TYPE STR_HEATER_FURNACE :
STRUCT
//INPUT
	Input_LOOP1_Process_Value	AT%I*	:	REAL	;
	Input_LOOP1_Alarm_Condition	AT%I*	:	UINT	;
	Input_LOOP1_Manipulated_Value_Control_Output	AT%I*	:	REAL	;
	Input_LOOP1_Controlling_Set_Point	AT%I*	:	REAL	;
	Input_LOOP1_Actual_Control_State	AT%I*	:	BOOL	;
	Input_LOOP1_Sensor_Error	AT%I*	:	BOOL	;
	Input_LOOP1_Actual_Control_Loop_Mode	AT%I*	:	BOOL	;
	Input_LOOP2_Process_Value	AT%I*	:	REAL	;
	Input_LOOP2_Alarm_Condition	AT%I*	:	UINT	;
	Input_LOOP2_Manipulated_Value_Control_Output	AT%I*	:	REAL	;
	Input_LOOP2_Controlling_Set_Point	AT%I*	:	REAL	;
	Input_LOOP2_Actual_Control_State	AT%I*	:	BOOL	;
	Input_LOOP2_Sensor_Error	AT%I*	:	BOOL	;
	Input_LOOP2_Actual_Control_Loop_Mode	AT%I*	:	BOOL	;
	Input_LOOP3_Process_Value	AT%I*	:	REAL	;
	Input_LOOP3_Alarm_Condition	AT%I*	:	UINT	;
	Input_LOOP3_Manipulated_Value_Control_Output	AT%I*	:	REAL	;
	Input_LOOP3_Controlling_Set_Point	AT%I*	:	REAL	;
	Input_LOOP3_Actual_Control_State	AT%I*	:	BOOL	;
	Input_LOOP3_Sensor_Error	AT%I*	:	BOOL	;
	Input_LOOP3_Actual_Control_Loop_Mode	AT%I*	:	BOOL	;
	Input_LOOP4_Process_Value	AT%I*	:	REAL	;
	Input_LOOP4_Alarm_Condition	AT%I*	:	UINT	;
	Input_LOOP4_Manipulated_Value_Control_Output	AT%I*	:	REAL	;
	Input_LOOP4_Controlling_Set_Point	AT%I*	:	REAL	;
	Input_LOOP4_Actual_Control_State	AT%I*	:	BOOL	;
	Input_LOOP4_Sensor_Error	AT%I*	:	BOOL	;
	Input_LOOP4_Actual_Control_Loop_Mode	AT%I*	:	BOOL	;
	Input_LOOP5_Process_Value	AT%I*	:	REAL	;
	Input_LOOP5_Alarm_Condition	AT%I*	:	UINT	;
	Input_LOOP5_Manipulated_Value_Control_Output	AT%I*	:	REAL	;
	Input_LOOP5_Controlling_Set_Point	AT%I*	:	REAL	;
	Input_LOOP5_Actual_Control_State	AT%I*	:	BOOL	;
	Input_LOOP5_Sensor_Error	AT%I*	:	BOOL	;
	Input_LOOP5_Actual_Control_Loop_Mode	AT%I*	:	BOOL	;
	Input_LOOP6_Process_Value	AT%I*	:	REAL	;
	Input_LOOP6_Alarm_Condition	AT%I*	:	UINT	;
	Input_LOOP6_Manipulated_Value_Control_Output	AT%I*	:	REAL	;
	Input_LOOP6_Controlling_Set_Point	AT%I*	:	REAL	;
	Input_LOOP6_Actual_Control_State	AT%I*	:	BOOL	;
	Input_LOOP6_Sensor_Error	AT%I*	:	BOOL	;
	Input_LOOP6_Actual_Control_Loop_Mode	AT%I*	:	BOOL	;
	Input_LOOP7_Process_Value	AT%I*	:	REAL	;
	Input_LOOP7_Alarm_Condition	AT%I*	:	UINT	;
	Input_LOOP7_Manipulated_Value_Control_Output	AT%I*	:	REAL	;
	Input_LOOP7_Controlling_Set_Point	AT%I*	:	REAL	;
	Input_LOOP7_Actual_Control_State	AT%I*	:	BOOL	;
	Input_LOOP7_Sensor_Error	AT%I*	:	BOOL	;
	Input_LOOP7_Actual_Control_Loop_Mode	AT%I*	:	BOOL	;
	Input_LOOP8_Process_Value	AT%I*	:	REAL	;
	Input_LOOP8_Alarm_Condition	AT%I*	:	UINT	;
	Input_LOOP8_Manipulated_Value_Control_Output	AT%I*	:	REAL	;
	Input_LOOP8_Controlling_Set_Point	AT%I*	:	REAL	;
	Input_LOOP8_Actual_Control_State	AT%I*	:	BOOL	;
	Input_LOOP8_Sensor_Error	AT%I*	:	BOOL	;
	Input_LOOP8_Actual_Control_Loop_Mode	AT%I*	:	BOOL	;
	Input_IO_Mod_1_PV	AT%I*	:	REAL	;
	Input_IO_Mod_2_PV	AT%I*	:	REAL	;
	Input_IO_Mod_3_PV	AT%I*	:	REAL	;
	Input_IO_Mod_4_PV	AT%I*	:	REAL	;
	Input_IO_Mod_5_PV	AT%I*	:	REAL	;
	Input_IO_Mod_6_PV	AT%I*	:	REAL	;
	Input_IO_Mod_7_PV	AT%I*	:	REAL	;
	Input_IO_Mod_9_PV	AT%I*	:	REAL	;
	Input_IO_Mod_10_PV	AT%I*	:	REAL	;
	Input_IO_Mod_11_PV	AT%I*	:	REAL	;
	Input_IO_Mod_12_PV	AT%I*	:	REAL	;
	Input_IO_Mod_13_PV	AT%I*	:	REAL	;
	Input_IO_Mod_14_PV	AT%I*	:	REAL	;
	Input_IO_Mod_15_PV	AT%I*	:	REAL	;
	Input_IO_Mod_18_PV	AT%I*	:	REAL	;
	Input_IO_Mod_19_PV	AT%I*	:	REAL	;
	Input_IO_Mod_20_PV	AT%I*	:	REAL	;
	Input_IO_Mod_21_PV	AT%I*	:	REAL	;
	Input_IO_Mod_22_PV	AT%I*	:	REAL	;
	Input_IO_Mod_23_PV	AT%I*	:	REAL	;
	Input_IO_Mod_1_SBrkOut	AT%I*	:	USINT	;
	Input_IO_Mod_2_SBrkOut	AT%I*	:	USINT	;
	Input_IO_Mod_3_SBrkOut	AT%I*	:	USINT	;
	Input_IO_Mod_4_SBrkOut	AT%I*	:	USINT	;
	Input_IO_Mod_5_SBrkOut	AT%I*	:	USINT	;
	Input_IO_Mod_6_SBrkOut	AT%I*	:	USINT	;
	Input_IO_Mod_7_SBrkOut	AT%I*	:	USINT	;
	Input_IO_Mod_9_SBrkOut	AT%I*	:	USINT	;
	Input_IO_Mod_10_SBrkOut	AT%I*	:	USINT	;
	Input_IO_Mod_11_SBrkOut	AT%I*	:	USINT	;
	Input_IO_Mod_12_SBrkOut	AT%I*	:	USINT	;
	Input_IO_Mod_13_SBrkOut	AT%I*	:	USINT	;
	Input_IO_Mod_14_SBrkOut	AT%I*	:	USINT	;
	Input_IO_Mod_15_SBrkOut	AT%I*	:	USINT	;
	Input_IO_Mod_18_SBrkOut	AT%I*	:	USINT	;
	Input_IO_Mod_19_SBrkOut	AT%I*	:	USINT	;
	Input_IO_Mod_20_SBrkOut	AT%I*	:	USINT	;
	Input_IO_Mod_21_SBrkOut	AT%I*	:	USINT	;
	Input_IO_Mod_22_SBrkOut	AT%I*	:	USINT	;
	Input_IO_Mod_23_SBrkOut	AT%I*	:	USINT	;
	Input_Math2_8_In2	AT%I*	:	REAL	;
	Input_Math2_12_In2	AT%I*	:	REAL	;
	Input_Math2_16_In2	AT%I*	:	REAL	;
	Input_Math2_20_In2	AT%I*	:	REAL	;
	Input_Math2_24_In2	AT%I*	:	REAL	;
	Input_Math2_28_In2	AT%I*	:	REAL	;
	Input_Loop_7_Setpoint	AT%I*	:	REAL	;
	Input_Loop_7_Setpoint_SPRateUp	AT%I*	:	REAL	;
	Input_Loop_7_Setpoint_SPRateDown	AT%I*	:	REAL	;
	Input_Loop_7_PID_Ch1PropBand	AT%I*	:	REAL	;
	Input_Loop_7_PID_IntegralTime	AT%I*	:	REAL	;
	Input_Loop_7_PID_DerivativeTime	AT%I*	:	REAL	;
	Input_Loop_1_Main_CascadeMode	AT%I*	:	USINT	;
	Input_Loop_1_Setpoint	AT%I*	:	REAL	;
	Input_Loop_1_Setpoint_SPRateUp	AT%I*	:	REAL	;
	Input_Loop_1_Setpoint_SPRateDown	AT%I*	:	REAL	;
	Input_Loop_1_Cascade_SecondaryLocalSP	AT%I*	:	REAL	;
	Input_Loop_1_Main_TC_Select	AT%I*	:	USINT	;
	Input_Loop_1_PrimaryPID_PrimaryPropBand	AT%I*	:	REAL	;
	Input_Loop_1_PrimaryPID_PrimaryIntegralTime	AT%I*	:	REAL	;
	Input_Loop_1_PrimaryPID_PrimaryDerivativeTime	AT%I*	:	REAL	;
	Input_Loop_1_PID_Ch1PropBand	AT%I*	:	REAL	;
	Input_Loop_1_PID_IntegralTime	AT%I*	:	REAL	;
	Input_Loop_1_PID_DerivativeTime	AT%I*	:	REAL	;
	Input_Loop_2_Main_CascadeMode	AT%I*	:	USINT	;
	Input_Loop_2_Setpoint	AT%I*	:	REAL	;
	Input_Loop_2_Setpoint_SPRateUp	AT%I*	:	REAL	;
	Input_Loop_2_Setpoint_SPRateDown	AT%I*	:	REAL	;
	Input_Loop_2_Cascade_SecondaryLocalSP	AT%I*	:	REAL	;
	Input_Loop_2_Main_TC_Select	AT%I*	:	USINT	;
	Input_Loop_2_PrimaryPID_PrimaryPropBand	AT%I*	:	REAL	;
	Input_Loop_2_PrimaryPID_PrimaryIntegralTime	AT%I*	:	REAL	;
	Input_Loop_2_PrimaryPID_PrimaryDerivativeTime	AT%I*	:	REAL	;
	Input_Loop_2_PID_Ch1PropBand	AT%I*	:	REAL	;
	Input_Loop_2_PID_IntegralTime	AT%I*	:	REAL	;
	Input_Loop_2_PID_DerivativeTime	AT%I*	:	REAL	;
	Input_Loop_3_Main_CascadeMode	AT%I*	:	USINT	;
	Input_Loop_3_Setpoint	AT%I*	:	REAL	;
	Input_Loop_3_Setpoint_SPRateUp	AT%I*	:	REAL	;
	Input_Loop_3_Setpoint_SPRateDown	AT%I*	:	REAL	;
	Input_Loop_3_Cascade_SecondaryLocalSP	AT%I*	:	REAL	;
	Input_Loop_3_Main_TC_Select	AT%I*	:	USINT	;
	Input_Loop_3_PrimaryPID_PrimaryPropBand	AT%I*	:	REAL	;
	Input_Loop_3_PrimaryPID_PrimaryIntegralTime	AT%I*	:	REAL	;
	Input_Loop_3_PrimaryPID_PrimaryDerivativeTime	AT%I*	:	REAL	;
	Input_Loop_3_PID_Ch1PropBand	AT%I*	:	REAL	;
	Input_Loop_3_PID_IntegralTime	AT%I*	:	REAL	;
	Input_Loop_3_PID_DerivativeTime	AT%I*	:	REAL	;
	Input_Loop_4_Main_CascadeMode	AT%I*	:	USINT	;
	Input_Loop_4_Setpoint	AT%I*	:	REAL	;
	Input_Loop_4_Setpoint_SPRateUp	AT%I*	:	REAL	;
	Input_Loop_4_Setpoint_SPRateDown	AT%I*	:	REAL	;
	Input_Loop_4_Cascade_SecondaryLocalSP	AT%I*	:	REAL	;
	Input_Loop_4_Main_TC_Select	AT%I*	:	USINT	;
	Input_Loop_4_PrimaryPID_PrimaryPropBand	AT%I*	:	REAL	;
	Input_Loop_4_PrimaryPID_PrimaryIntegralTime	AT%I*	:	REAL	;
	Input_Loop_4_PrimaryPID_PrimaryDerivativeTime	AT%I*	:	REAL	;
	Input_Loop_4_PID_Ch1PropBand	AT%I*	:	REAL	;
	Input_Loop_4_PID_IntegralTime	AT%I*	:	REAL	;
	Input_Loop_4_PID_DerivativeTime	AT%I*	:	REAL	;
	Input_Loop_5_Main_CascadeMode	AT%I*	:	USINT	;
	Input_Loop_5_Setpoint	AT%I*	:	REAL	;
	Input_Loop_5_Setpoint_SPRateUp	AT%I*	:	REAL	;
	Input_Loop_5_Setpoint_SPRateDown	AT%I*	:	REAL	;
	Input_Loop_5_Cascade_SecondaryLocalSP	AT%I*	:	REAL	;
	Input_Loop_5_Main_TC_Select	AT%I*	:	USINT	;
	Input_Loop_5_PrimaryPID_PrimaryPropBand	AT%I*	:	REAL	;
	Input_Loop_5_PrimaryPID_PrimaryIntegralTime	AT%I*	:	REAL	;
	Input_Loop_5_PrimaryPID_PrimaryDerivativeTime	AT%I*	:	REAL	;
	Input_Loop_5_PID_Ch1PropBand	AT%I*	:	REAL	;
	Input_Loop_5_PID_IntegralTime	AT%I*	:	REAL	;
	Input_Loop_5_PID_DerivativeTime	AT%I*	:	REAL	;
	Input_Loop_6_Main_CascadeMode	AT%I*	:	USINT	;
	Input_Loop_6_Setpoint	AT%I*	:	REAL	;
	Input_Loop_6_Setpoint_SPRateUp	AT%I*	:	REAL	;
	Input_Loop_6_Setpoint_SPRateDown	AT%I*	:	REAL	;
	Input_Loop_6_Cascade_SecondaryLocalSP	AT%I*	:	REAL	;
	Input_Loop_6_Main_TC_Select	AT%I*	:	USINT	;
	Input_Loop_6_PrimaryPID_PrimaryPropBand	AT%I*	:	REAL	;
	Input_Loop_6_PrimaryPID_PrimaryIntegralTime	AT%I*	:	REAL	;
	Input_Loop_6_PrimaryPID_PrimaryDerivativeTime	AT%I*	:	REAL	;
	Input_Loop_6_PID_Ch1PropBand	AT%I*	:	REAL	;
	Input_Loop_6_PID_IntegralTime	AT%I*	:	REAL	;
	Input_Loop_6_PID_DerivativeTime	AT%I*	:	REAL	;
	Input_Instrument_Diagnostics_ForceStandby	AT%I*	:	USINT	;
	
//OUTPUT
	Output_LOOP1_Target_Set_Point	AT%Q*	:	REAL	;
	Output_LOOP1_Clear_Alarms	AT%Q*	:	UINT	;
	Output_LOOP1_Forced_MV	AT%Q*	:	REAL	;
	Output_LOOP1_Control_Mode	AT%Q*	:	BOOL	;
	Output_LOOP1_Control_State	AT%Q*	:	BOOL	;
	Output_LOOP2_Target_Set_Point	AT%Q*	:	REAL	;
	Output_LOOP2_Clear_Alarms	AT%Q*	:	UINT	;
	Output_LOOP2_Forced_MV	AT%Q*	:	REAL	;
	Output_LOOP2_Control_Mode	AT%Q*	:	BOOL	;
	Output_LOOP2_Control_State	AT%Q*	:	BOOL	;
	Output_LOOP3_Target_Set_Point	AT%Q*	:	REAL	;
	Output_LOOP3_Clear_Alarms	AT%Q*	:	UINT	;
	Output_LOOP3_Forced_MV	AT%Q*	:	REAL	;
	Output_LOOP3_Control_Mode	AT%Q*	:	BOOL	;
	Output_LOOP3_Control_State	AT%Q*	:	BOOL	;
	Output_LOOP4_Target_Set_Point	AT%Q*	:	REAL	;
	Output_LOOP4_Clear_Alarms	AT%Q*	:	UINT	;
	Output_LOOP4_Forced_MV	AT%Q*	:	REAL	;
	Output_LOOP4_Control_Mode	AT%Q*	:	BOOL	;
	Output_LOOP4_Control_State	AT%Q*	:	BOOL	;
	Output_LOOP5_Target_Set_Point	AT%Q*	:	REAL	;
	Output_LOOP5_Clear_Alarms	AT%Q*	:	UINT	;
	Output_LOOP5_Forced_MV	AT%Q*	:	REAL	;
	Output_LOOP5_Control_Mode	AT%Q*	:	BOOL	;
	Output_LOOP5_Control_State	AT%Q*	:	BOOL	;
	Output_LOOP6_Target_Set_Point	AT%Q*	:	REAL	;
	Output_LOOP6_Clear_Alarms	AT%Q*	:	UINT	;
	Output_LOOP6_Forced_MV	AT%Q*	:	REAL	;
	Output_LOOP6_Control_Mode	AT%Q*	:	BOOL	;
	Output_LOOP6_Control_State	AT%Q*	:	BOOL	;
	Output_LOOP7_Target_Set_Point	AT%Q*	:	REAL	;
	Output_LOOP7_Clear_Alarms	AT%Q*	:	UINT	;
	Output_LOOP7_Forced_MV	AT%Q*	:	REAL	;
	Output_LOOP7_Control_Mode	AT%Q*	:	BOOL	;
	Output_LOOP7_Control_State	AT%Q*	:	BOOL	;
	Output_LOOP8_Target_Set_Point	AT%Q*	:	REAL	;
	Output_LOOP8_Clear_Alarms	AT%Q*	:	UINT	;
	Output_LOOP8_Forced_MV	AT%Q*	:	REAL	;
	Output_LOOP8_Control_Mode	AT%Q*	:	BOOL	;
	Output_LOOP8_Control_State	AT%Q*	:	BOOL	;
	Output_Math2_8_In2	AT%Q*	:	REAL	;
	Output_Math2_12_In2	AT%Q*	:	REAL	;
	Output_Math2_16_In2	AT%Q*	:	REAL	;
	Output_Math2_20_In2	AT%Q*	:	REAL	;
	Output_Math2_24_In2	AT%Q*	:	REAL	;
	Output_Math2_28_In2	AT%Q*	:	REAL	;
	Output_Loop_7_Setpoint_SPRateUp	AT%Q*	:	REAL	;
	Output_Loop_7_Setpoint_SPRateDown	AT%Q*	:	REAL	;
	Output_Loop_7_PID_Ch1PropBand	AT%Q*	:	REAL	;
	Output_Loop_7_PID_IntegralTime	AT%Q*	:	REAL	;
	Output_Loop_7_PID_DerivativeTime	AT%Q*	:	REAL	;
	Output_Loop_1_Main_CascadeMode	AT%Q*	:	USINT	;
	Output_Loop_1_Setpoint_SPRateUp	AT%Q*	:	REAL	;
	Output_Loop_1_Setpoint_SPRateDown	AT%Q*	:	REAL	;
	Output_Loop_1_Cascade_SecondaryLocalSP	AT%Q*	:	REAL	;
	Output_Loop_1_Main_TC_Select	AT%Q*	:	USINT	;
	Output_Loop_1_PrimaryPID_PrimaryPropBand	AT%Q*	:	REAL	;
	Output_Loop_1_PrimaryPID_PrimaryIntegralTime	AT%Q*	:	REAL	;
	Output_Loop_1_PrimaryPID_PrimaryDerivativeTime	AT%Q*	:	REAL	;
	Output_Loop_1_PID_Ch1PropBand	AT%Q*	:	REAL	;
	Output_Loop_1_PID_IntegralTime	AT%Q*	:	REAL	;
	Output_Loop_1_PID_DerivativeTime	AT%Q*	:	REAL	;
	Output_Loop_2_Main_CascadeMode	AT%Q*	:	USINT	;
	Output_Loop_2_Setpoint_SPRateUp	AT%Q*	:	REAL	;
	Output_Loop_2_Setpoint_SPRateDown	AT%Q*	:	REAL	;
	Output_Loop_2_Cascade_SecondaryLocalSP	AT%Q*	:	REAL	;
	Output_Loop_2_Main_TC_Select	AT%Q*	:	USINT	;
	Output_Loop_2_PrimaryPID_PrimaryPropBand	AT%Q*	:	REAL	;
	Output_Loop_2_PrimaryPID_PrimaryIntegralTime	AT%Q*	:	REAL	;
	Output_Loop_2_PrimaryPID_PrimaryDerivativeTime	AT%Q*	:	REAL	;
	Output_Loop_2_PID_Ch1PropBand	AT%Q*	:	REAL	;
	Output_Loop_2_PID_IntegralTime	AT%Q*	:	REAL	;
	Output_Loop_2_PID_DerivativeTime	AT%Q*	:	REAL	;
	Output_Loop_3_Main_CascadeMode	AT%Q*	:	USINT	;
	Output_Loop_3_Setpoint_SPRateUp	AT%Q*	:	REAL	;
	Output_Loop_3_Setpoint_SPRateDown	AT%Q*	:	REAL	;
	Output_Loop_3_Cascade_SecondaryLocalSP	AT%Q*	:	REAL	;
	Output_Loop_3_Main_TC_Select	AT%Q*	:	USINT	;
	Output_Loop_3_PrimaryPID_PrimaryPropBand	AT%Q*	:	REAL	;
	Output_Loop_3_PrimaryPID_PrimaryIntegralTime	AT%Q*	:	REAL	;
	Output_Loop_3_PrimaryPID_PrimaryDerivativeTime	AT%Q*	:	REAL	;
	Output_Loop_3_PID_Ch1PropBand	AT%Q*	:	REAL	;
	Output_Loop_3_PID_IntegralTime	AT%Q*	:	REAL	;
	Output_Loop_3_PID_DerivativeTime	AT%Q*	:	REAL	;
	Output_Loop_4_Main_CascadeMode	AT%Q*	:	USINT	;
	Output_Loop_4_Setpoint_SPRateUp	AT%Q*	:	REAL	;
	Output_Loop_4_Setpoint_SPRateDown	AT%Q*	:	REAL	;
	Output_Loop_4_Cascade_SecondaryLocalSP	AT%Q*	:	REAL	;
	Output_Loop_4_Main_TC_Select	AT%Q*	:	USINT	;
	Output_Loop_4_PrimaryPID_PrimaryPropBand	AT%Q*	:	REAL	;
	Output_Loop_4_PrimaryPID_PrimaryIntegralTime	AT%Q*	:	REAL	;
	Output_Loop_4_PrimaryPID_PrimaryDerivativeTime	AT%Q*	:	REAL	;
	Output_Loop_4_PID_Ch1PropBand	AT%Q*	:	REAL	;
	Output_Loop_4_PID_IntegralTime	AT%Q*	:	REAL	;
	Output_Loop_4_PID_DerivativeTime	AT%Q*	:	REAL	;
	Output_Loop_5_Main_CascadeMode	AT%Q*	:	USINT	;
	Output_Loop_5_Setpoint_SPRateUp	AT%Q*	:	REAL	;
	Output_Loop_5_Setpoint_SPRateDown	AT%Q*	:	REAL	;
	Output_Loop_5_Cascade_SecondaryLocalSP	AT%Q*	:	REAL	;
	Output_Loop_5_Main_TC_Select	AT%Q*	:	USINT	;
	Output_Loop_5_PrimaryPID_PrimaryPropBand	AT%Q*	:	REAL	;
	Output_Loop_5_PrimaryPID_PrimaryIntegralTime	AT%Q*	:	REAL	;
	Output_Loop_5_PrimaryPID_PrimaryDerivativeTime	AT%Q*	:	REAL	;
	Output_Loop_5_PID_Ch1PropBand	AT%Q*	:	REAL	;
	Output_Loop_5_PID_IntegralTime	AT%Q*	:	REAL	;
	Output_Loop_5_PID_DerivativeTime	AT%Q*	:	REAL	;
	Output_Loop_6_Main_CascadeMode	AT%Q*	:	USINT	;
	Output_Loop_6_Setpoint_SPRateUp	AT%Q*	:	REAL	;
	Output_Loop_6_Setpoint_SPRateDown	AT%Q*	:	REAL	;
	Output_Loop_6_Cascade_SecondaryLocalSP	AT%Q*	:	REAL	;
	Output_Loop_6_Main_TC_Select	AT%Q*	:	USINT	;
	Output_Loop_6_PrimaryPID_PrimaryPropBand	AT%Q*	:	REAL	;
	Output_Loop_6_PrimaryPID_PrimaryIntegralTime	AT%Q*	:	REAL	;
	Output_Loop_6_PrimaryPID_PrimaryDerivativeTime	AT%Q*	:	REAL	;
	Output_Loop_6_PID_Ch1PropBand	AT%Q*	:	REAL	;
	Output_Loop_6_PID_IntegralTime	AT%Q*	:	REAL	;
	Output_Loop_6_PID_DerivativeTime	AT%Q*	:	REAL	;
	Output_Instrument_Diagnostics_ForceStandby	AT%Q*	:	USINT	;






END_STRUCT
END_TYPE
